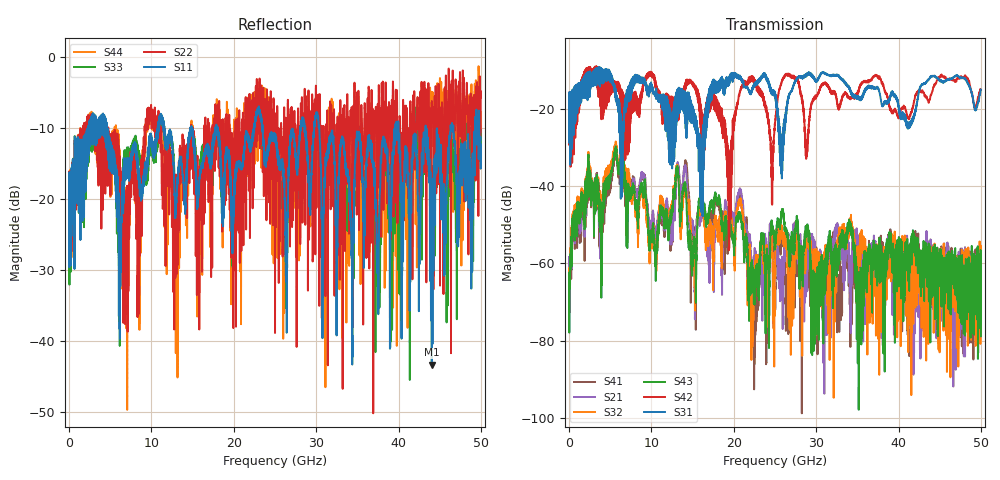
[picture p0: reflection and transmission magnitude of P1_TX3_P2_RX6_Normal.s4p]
!Keysight Technologies,N5225B,MY57041031,A.13.20.10
!Date: Friday, May 31, 2019 11:36:55
!Correction: S11(Full 4 Port(1,2,3,4))
!S12(Full 4 Port(1,2,3,4))
!S13(Full 4 Port(1,2,3,4))
!S14(Full 4 Port(1,2,3,4))
!S21(Full 4 Port(1,2,3,4))
!S22(Full 4 Port(1,2,3,4))
!S23(Full 4 Port(1,2,3,4))
!S24(Full 4 Port(1,2,3,4))
!S31(Full 4 Port(1,2,3,4))
!S32(Full 4 Port(1,2,3,4))
!S33(Full 4 Port(1,2,3,4))
!S34(Full 4 Port(1,2,3,4))
!S41(Full 4 Port(1,2,3,4))
!S42(Full 4 Port(1,2,3,4))
!S43(Full 4 Port(1,2,3,4))
!S44(Full 4 Port(1,2,3,4))
!S4P File: Measurements: <S11,S12,S13,S14>,
!<S21,S22,S23,S24>,
!<S31,S32,S33,S34>,
!<S41,S42,S43,S44>:
# Hz S  dB  R 50.0
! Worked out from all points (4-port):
!   5000 points, 10 MHz to 50 GHz, reference 50 ohm
!   strongest paths, dB at 10 MHz, 12.51 GHz, 25.01 GHz, 37.51 GHz, 50 GHz:
!     S31: -19.4, -27.1, -15.7, -14.5, -15.0
!     S42: -19.4, -16.9, -23.6, -11.6, -15.0
!     S43: -62.4, -46.7, -54.6, -59.7, -78.9
!     S32: -64.9, -45.6, -58.7, -71.9, -69.4
!     S21: -58.3, -53.0, -58.2, -60.0, -66.3
!     S41: -63.2, -52.5, -63.9, -58.8, -73.5
!   lowest |S11| = -43.3 dB at 44.03 GHz (marker M1), VSWR 1.01, Z = 50.1 + j0.67 ohm
!   |S11| at or under -10 dB: 4.66 GHz to 10.77 GHz (6.106 GHz wide, 79.2 % of centre); 23.49 GHz to 28.08 GHz (4.584 GHz wide, 17.8 % of centre); 30.37 GHz to 39.61 GHz (9.239 GHz wide, 26.4 % of centre)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
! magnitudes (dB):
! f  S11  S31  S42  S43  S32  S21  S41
! 10 MHz  -19.6  -19.4  -19.4  -62.4  -64.9  -58.3  -63.2
! 5.61 GHz  -16.5  -14.7  -14.7  -31.1  -29.7  -31.1  -32.6
! 15.17 GHz  -12.4  -23.3  -14.1  -53.1  -57.2  -52.8  -51.5
! 20.73 GHz  -15.3  -11.3  -15.5  -47.0  -43.3  -40.8  -42.4
! 22.66 GHz  -9.0  -13.5  -13.5  -62.0  -59.6  -58.3  -77.4
! 44.03 GHz  -43.3  -11.4  -15.9  -59.1  -65.6  -56.4  -63.1
! 50 GHz  -12.3  -15.0  -15.0  -78.9  -69.4  -66.3  -73.5
